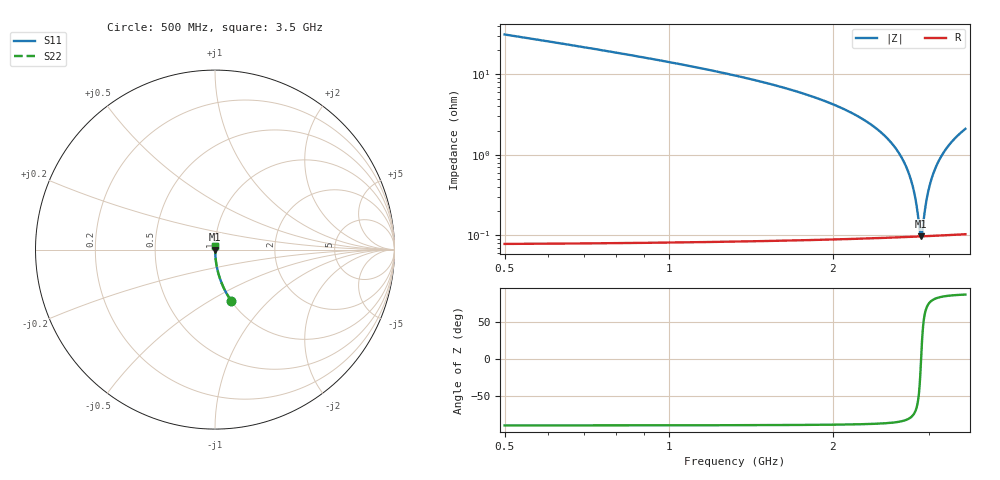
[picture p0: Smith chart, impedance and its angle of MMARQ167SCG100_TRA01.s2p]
! MMARQ167SCG100_TRA01  S-PARAMETER MODEL  ( General Type )
! Model Generated by TAIYO YUDEN Corporation (http://www.ty-top.com)
! Version 1.0
! TAIYO YUDEN Control No. 150305
! Copyright(c) 2015 TAIYO YUDEN CO.,LTD. All Rights Reserved.
! Product Description (link to TY-COMPAS)
! https://ds.yuden.co.jp/TYCOMPAS/or/detail?pn=MMARQ167SCG100GTRA01&u=M
! Products Name : Multilayer Ceramic Capacitors
! Characteristics :
!  Capacitance : 10 pF , Rated Voltage : 250V , TCC : CG / C0G
!  Case Size : 1.6 x 0.8 / 0.063 x 0.031 [mm/inch] , Thickness : 0.7 / 0.028 [mm/inch]
!  (Conditions: Temperature = 25 degC , DC Bias Current/Voltage = 0A / 0V)
! External Node Assignments :
!  1  o---| |---o  2
! GND o---------o GND
! Frequency Range : 500MHz  -  3.5GHz  [ 401 STEP ]
# MHz S RI R 50
! Freq[MHz].  S11 Real  S11 Imag  S21 Real  S21 Imag  S12 Real  S12 Imag  S22 Real  S22 Imag
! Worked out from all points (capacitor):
!   401 points, 500 MHz to 3.5 GHz, reference 50 ohm
!   read as one part in series: C = 9.81 pF near 515 MHz
!   lowest |Z| = 96.9 mohm at 2.9 GHz (marker M1)
!   series resonance near 2.903 GHz, so ESL is about 310 pH
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500  0.0907 -0.286  0.9093 0.286  0.9093 0.286  0.0907 -0.286
725  0.0428 -0.2006  0.9572 0.2006  0.9572 0.2006  0.0428 -0.2006
1002.5  0.0207 -0.1394  0.9793 0.1394  0.9793 0.1394  0.0207 -0.1394
1505  0.007 -0.0782  0.993 0.0782  0.993 0.0782  0.007 -0.0782
2000  0.00269 -0.0424  0.9973 0.0424  0.9973 0.0424  0.00269 -0.0424
2285  0.00163 -0.0269  0.9984 0.0269  0.9984 0.0269  0.00163 -0.0269
2502.5  0.0012 -0.0166  0.9988 0.0166  0.9988 0.0166  0.0012 -0.0166
2652.5  0.00104 -0.0101  0.999 0.0101  0.999 0.0101  0.00104 -0.0101
2712.5  0.001 -0.00756  0.999 0.00756  0.999 0.00756  0.001 -0.00756
2757.5  0.000981 -0.00573  0.999 0.00573  0.999 0.00573  0.000981 -0.00573
2795  0.00097 -0.00422  0.999 0.00422  0.999 0.00422  0.00097 -0.00422
2825  0.000964 -0.00303  0.999 0.00303  0.999 0.00303  0.000964 -0.00303
2847.5  0.000962 -0.00214  0.999 0.00214  0.999 0.00214  0.000962 -0.00214
2885  0.000961 -0.000685  0.999 0.000685  0.999 0.000685  0.000961 -0.000685
2900  0.000963 -0.000107  0.999 0.000107  0.999 0.000107  0.000963 -0.000107
2915  0.000964 0.000468  0.999 -0.000468  0.999 -0.000468  0.000964 0.000468
2960  0.000973 0.00218  0.999 -0.00218  0.999 -0.00218  0.000973 0.00218
3005  0.000988 0.00386  0.999 -0.00386  0.999 -0.00386  0.000988 0.00386
3080  0.00102 0.00661  0.999 -0.00661  0.999 -0.00661  0.00102 0.00661
3185  0.0011 0.0104  0.9989 -0.0104  0.9989 -0.0104  0.0011 0.0104
3327.5  0.00124 0.0153  0.9988 -0.0153  0.9988 -0.0153  0.00124 0.0153
3500  0.00147 0.021  0.9985 -0.021  0.9985 -0.021  0.00147 0.021
